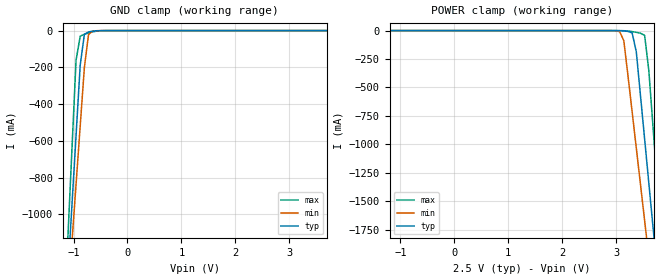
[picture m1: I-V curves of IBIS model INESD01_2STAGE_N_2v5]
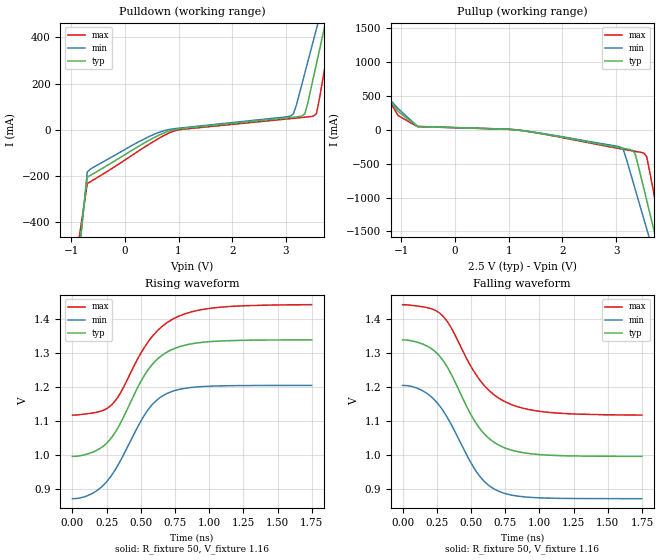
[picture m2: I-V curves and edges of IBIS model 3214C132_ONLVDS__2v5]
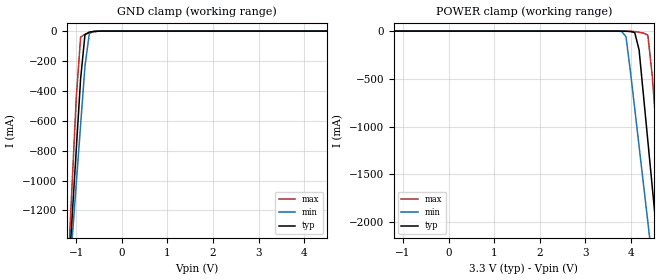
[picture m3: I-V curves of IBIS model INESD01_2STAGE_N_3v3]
|   This file is an IBIS representation of the   |
|   Integrated Device Technology, Inc.   |
|   ICS844021-01   |
|   FEMTOCLOCKS CRYSTAL-TO-LVDS CLOCK GENERATOR   |
[IBIS Ver]   4.1
[File name]   844021_01.ibs
[File Rev]   1.0
[Date]   29 Jul 2009 | Last modified
|   Sep  12 2007 | Generated
[Source]   Originated at Integrated Device Technology, Inc.
[Disclaimer]
IDT hereby grants the user of this IBIS model a non-exclusive,
nontransferable license to use this IBIS model under the following terms.
Before using this IBIS model, the user should read this license.
If the user does not accept these terms,  the IBIS model should be
returned to IDT within 30 days.
   The user is granted this license only to use the IBIS model and
is not granted rights to sell, load, rent, lease or license the IBIS
model in whole or in part, or in modified form to anyone other than
user. User may modify the IBIS model to suit its specific
applications but rights to derivative works and such modifications
shall belong to IDT.
   This IBIS model is provided on an "AS IS" basis and IDT makes
absolutely no warranty with respect to the information contained
herein. IDT DISCLAIMS AND CUSTOMER WAIVES ALL WARRANTIES, EXPRESS
OR IMPLIED, INCLUDING WARRANTIES OF MERCHANTABILITY OR FITNESS FOR
A PARTICULAR PURPOSE. The entire risk as to quality and performance
is with the Customer. ACCORDINGLY, IN NO EVENT SHALL THE COMPANY BE
LIABLE FOR ANY DAMAGES, WHETHER IN CONTRACT OR TORT,INCLUDING ANY
LOST PROFITS OR OTHER INCIDENTAL, CONSEQUENTIAL, EXEMPLARY, OR
PUNITIVE DAMAGES ARISING OUT OF THE USE OR APPLICATION OF THE IBIS
model provided in this package. Further, IDT reserves the right to
make changes without notice to any product herein to improve
reliability, function, or design. IDT does not convey any license
under patent rights or any other intellectual property rights,
including those of third parties.
   IDT is not obligated to provide maintenance or support
for the licensed IBIS model.
[Copyright]   Copyright 2007 by Integrated Device Technology, Inc.
[Component]   ICS844021G-01
[Manufacturer] Integrated Device Technology, Inc.
[Package]
|TSSOP 8 Lead
|   typ   min   max
R_pkg   52.5m   48.8m   56.2m
L_pkg   1.381nH   1.275nH   1.486nH
C_pkg   0.236pF   0.230pF   0.242pF
[Pin] signal_name  model_name   R_pin   L_pin   C_pin
1   VDDA   POWER   56.2m   1.486n   0.242p
2   GND   GND   48.8m   1.275n   0.230p
3   XTAL_OUT   NC   48.8m   1.275n   0.230p
4   XTAL_IN   NC   56.2m   1.468n   0.242p
5   OE   INESD01_2STAGE_N   56.2m   1.486n   0.242p
6   nQ   3214C132_ONLVDS_   48.8m   1.275n   0.230p
7   Q   3214C132_ONLVDS_   48.8m   1.275n   0.230p
8   VDD   POWER   56.2m   1.468n   0.242p
[Diff Pin]  inv_pin  vdiff tdelay_typ tdelay_min  tdelay_max
7   6   NA   0  0  0
[Model Selector] INESD01_2STAGE_N
INESD01_2STAGE_N_2v5  Buffer selection for 2v5
INESD01_2STAGE_N_3v3  Buffer selection for 3v3
[Model Selector] 3214C132_ONLVDS_
3214C132_ONLVDS__2v5  Buffer selection for 2v5
3214C132_ONLVDS__3v3  Buffer selection for 3v3
| Models and submodels in the file (4): INESD01_2STAGE_N_2v5 (Input), 3214C132_ONLVDS__2v5 (Output), INESD01_2STAGE_N_3v3 (Input), 3214C132_ONLVDS__3v3 (Output)
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[Model] INESD01_2STAGE_N_2v5
Model_type   Input
Polarity   Non-Inverting
Vinl = 0.7V
Vinh = 1.7V
|   typ   min   max
C_comp   2pF   1.5pF   2.5pF
|   typ   min   max
[Voltage range]  2.5V   2.375V   2.625V
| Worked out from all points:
|   GND clamp passes 1 mA (typ) near -0.56 V on its own axis
[GND_clamp]
|Voltage   I(typ)   I(min)   I(max)
-2.5V     -8.269A    -7.245A    -9.986A
-1.108V   -1.338A    -1.475A    -1.143A
-1.031V   -954.2mA   -1.155A    -652.3mA
-953.6mV  -570.3mA   -836.3mA   -161.2mA
-876.3mV  -186.9mA   -517.8mA   -30.2mA
-799mV    -20.08mA   -199.8mA   -19.87mA
-721.6mV  -7.049mA   -21.01mA   -12.75mA
-644.3mV  -3.148mA   -2.874mA   -6.745mA
-489.7mV  -290.5uA   -172.1uA   -617.5uA
5V        48.47uA    63.64uA    35.68uA
[POWER_clamp]
|Voltage   I(typ)   I(min)   I(max)
-2.5V     48.47uA    60.61uA    37.56uA
3.067V    -1.084mA   -9.257mA   -231.1uA
3.144V    -3.149mA   -87.7mA    -1.112mA
3.299V    -20.08mA   -714.1mA   -8.879mA
3.376V    -186.9mA   -1.033A    -15.37mA
3.454V    -570.3mA   -1.352A    -22.95mA
3.531V    -954.2mA   -1.672A    -42.3mA
3.608V    -1.338A    -1.991A    -349.4mA
3.686V    -1.723A    -2.311A    -840.5mA
3.763V    -2.108A    -2.632A    -1.332A
3.84V     -2.492A    -2.952A    -1.823A
5V        -8.269A    -7.765A    -9.192A
[Model] 3214C132_ONLVDS__2v5
Model_type   Output
Polarity   Non-Inverting
|   typ   min   max
C_comp   2pF   1.5pF   2.5pF
Vmeas = 1.16V
Rref = 50
Cref = 0
Vref = 1.16V
|   typ   min   max
[Voltage range]   2.5V   2.375V   2.625V
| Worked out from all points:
|   slope of the pulldown table from 0 to 0.375 V, typ, clamps not added: 7.16 ohm
|   slope of the pullup table from 0 to 0.375 V, typ, clamps not added: 42.3 ohm
|   rising waveform, R_fixture 50, V_fixture 1.16: 20-80 % time 282ps typ, 280ps min, 302ps max; typ from 0.996 V to 1.34 V
|   falling waveform, R_fixture 50, V_fixture 1.16: 20-80 % time 283ps typ, 280ps min, 302ps max; typ from 1.34 V to 0.996 V
[Pulldown]
|Voltage   I (typ)   I (min)   I (max)
-2.5V     -5.621A    -4.951A    -6.736A
-1.06V    -934.3mA   -1.024A    -786.2mA
-699mV    -204mA     -181.3mA   -231.6mA
597.3mV   -27.26mA   -14.45mA   -41.66mA
3.082V    53.06mA    59.59mA    48.35mA
3.352V    69.36mA    245.7mA    54.57mA
3.514V    229mA      388.4mA    59.39mA
3.568V    285.7mA    436mA      70.08mA
3.73V     456.2mA    579mA      276.8mA
3.838V    570mA      674.4mA    421.1mA
3.892V    626.9mA    722.2mA    493.4mA
5V        1.798A     1.703A     1.979A
[Pullup]
|Voltage   I (typ)   I (min)   I (max)
-2.5V     1.791A     1.586A     2.14A
-2.14V    1.41A      1.267A     1.657A
-1.06V    270.5mA    312.2mA    210.3mA
-700mV    49.14mA    52.45mA    47.43mA
1.137V    -1.538mA   -1.006mA   752.2uA
3.082V    -266.5mA   -256.6mA   -279.9mA
3.352V    -346.7mA   -870.6mA   -317.4mA
3.514V    -862.6mA   -1.313A    -342.6mA
3.568V    -1.038A    -1.46A     -393.8mA
3.73V     -1.566A    -1.902A    -1.054A
3.838V    -1.918A    -2.197A    -1.5A
5V        -5.7A      -5.366A    -6.3A
[Ramp]
|   typ   min   max
dV/dt_r   0.274/0.46n   0.266/0.44n   0.259/0.494n
dV/dt_f   0.274/0.46n   0.266/0.44n   0.259/0.494n
R_load =   50.0000
[Rising Waveform]
R_fixture = 50
V_fixture = 1.16   |Vcc_typ
V_fixture_min = 1.05 |Vcc_min
V_fixture_max = 1.27 |Vcc_max
C_fixture = 0.0p
| Time   typ   min   max
0s        995.6mV    871.2mV    1.117V
159.4ps   1.01V      889.9mV    1.124V
289ps     1.052V     941.5mV    1.148V
353.9ps   1.095V     984.9mV    1.184V
539.5ps   1.242V     1.125V     1.325V
609.6ps   1.277V     1.159V     1.36V
690.2ps   1.302V     1.18V      1.389V
828.6ps   1.323V     1.196V     1.416V
1.02ns    1.334V     1.202V     1.432V
1.748ns   1.338V     1.204V     1.442V
[Falling Waveform]
R_fixture = 50
V_fixture = 1.16   |Vcc_typ
V_fixture_min = 1.05 |Vcc_min
V_fixture_max = 1.27 |Vcc_max
C_fixture = 0.0p
| Time   typ   min   max
0s        1.338V     1.205V     1.442V
159.4ps   1.324V     1.186V     1.435V
289ps     1.282V     1.134V     1.411V
353.9ps   1.239V     1.091V     1.375V
539.5ps   1.092V     950.8mV    1.235V
609.6ps   1.057V     917.3mV    1.199V
691.9ps   1.032V     895.1mV    1.17V
832.1ps   1.01V      879.4mV    1.143V
1.02ns    1.001V     873.5mV    1.127V
1.748ns   995.8mV    871.3mV    1.117V
[Model] INESD01_2STAGE_N_3v3
Model_type   Input
Polarity   Non-Inverting
Vinl = 0.8V
Vinh = 2.0V
|   typ   min   max
C_comp   2pF   1.5pF   2.5pF
|   typ   min   max
[Voltage range]  3.3V   3.15V   3.45V
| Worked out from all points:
|   GND clamp passes 1 mA (typ) near -0.55 V on its own axis
[GND_clamp]
|Voltage   I(typ)   I(min)   I(max)
-3.3V     -12.25A    -10.57A    -15.07A
-1.191V   -1.749A    -1.815A    -1.667A
-1.095V   -1.272A    -1.419A    -1.058A
-999mV    -795.5mA   -1.023A    -449.3mA
-903.1mV  -319.8mA   -628.1mA   -40.47mA
-807.2mV  -23.98mA   -233.7mA   -20.7mA
-711.3mV  -6.373mA   -15.69mA   -11.88mA
-615.5mV  -2.208mA   -1.554mA   -4.927mA
-519.6mV  -502.9uA   -282.7uA   -1.127mA
6V        52.35uA    69.46uA    38.08uA
[POWER_clamp]
|Voltage   I(typ)   I(min)   I(max)
-3.3V     63.98uA    80.01uA    49.58uA
3.795V    -332uA     -4.132mA   -63.8uA
3.891V    -1.568mA   -57.73mA   -179.8uA
3.987V    -4.988mA   -416.2mA   -1.17mA
4.082V    -14.84mA   -811mA     -5.045mA
4.178V    -197.1mA   -1.206A    -12.05mA
4.37V     -1.149A    -1.999A    -41.75mA
4.466V    -1.626A    -2.396A    -462.1mA
4.562V    -2.102A    -2.793A    -1.071A
4.658V    -2.58A     -3.19A     -1.68A
4.754V    -3.057A    -3.588A    -2.29A
6V        -9.266A    -8.761A    -10.21A
